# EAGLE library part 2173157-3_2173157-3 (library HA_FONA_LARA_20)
Conn Micro USB 2.0 Type B RCP 5 POS 0.65mm Solder RA SMD 5 Terminal 1 Port T/R Check prices
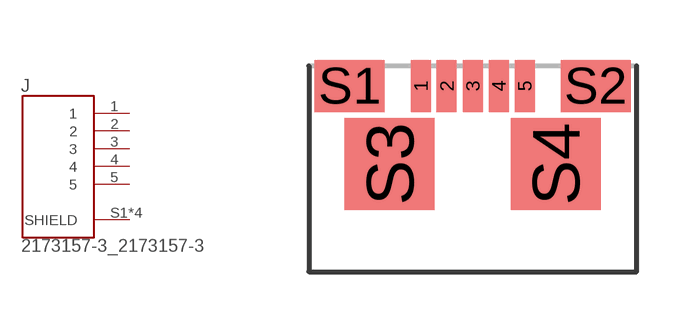
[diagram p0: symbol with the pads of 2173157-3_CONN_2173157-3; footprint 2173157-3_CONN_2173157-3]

Designator prefix J

## 2173157-3_2173157-3 (AVAILABILITY: Good; CENTERLINE_PITCH: .65 mm[.025 in]; COMMENT: 2173157-3; DESCRIPTION: Conn Micro USB 2.0 Type B RCP 5 POS 0.65mm Solder RA SMD 5 Terminal 1 Port T/R; EU_ROHS_COMPLIANCE: Compliant; MF: TE Connectivity; MP: 2173157-3; NUMBER_OF_POSITIONS: 5; PACKAGE: None; PRICE: None; PRODUCT_TYPE: Connector; PURCHASE-URL: https://pricing.snapeda.com/search/part/2173157-3/?ref=eda)  [2173157-3_CONN_2173157-3]
1  1  pas
2  2  pas
3  3  pas
4  4  pas
5  5  pas
S1  SHIELD  pas
S2  SHIELD  pas
S3  SHIELD  pas
S4  SHIELD  pas

## Footprint 2173157-3_CONN_2173157-3 (pad centres in mm)
smd 0.5 x 1.3: 1 -1.3,0; 2 -0.65,0; 3 0,0; 4 0.65,0; 5 1.3,0
smd 1.75 x 1.3: S1 -3.075,0; S2 3.075,0
smd 2.25 x 2.3: S3 -2.075,-1.95; S4 2.075,-1.95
